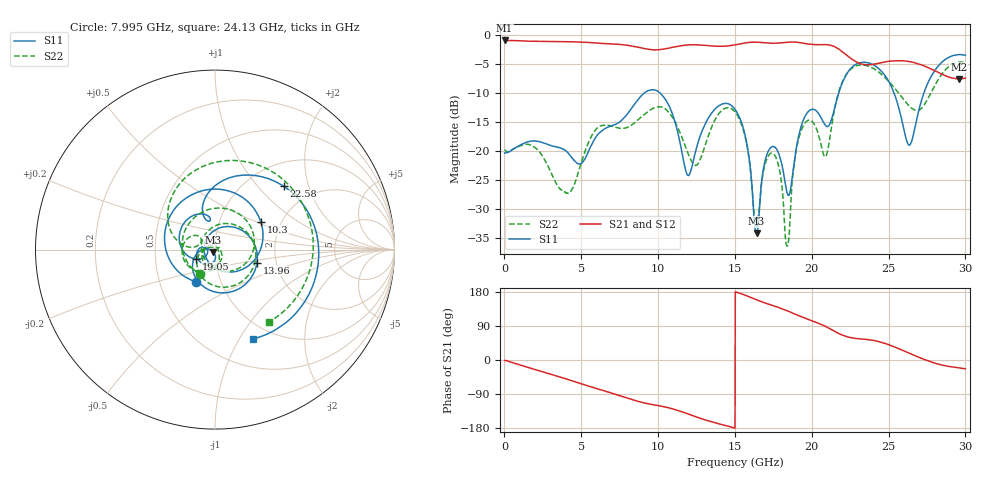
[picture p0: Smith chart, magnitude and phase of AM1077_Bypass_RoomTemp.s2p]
# Hz S DB R 50.0
!freq dBS11 angS11 dBS21 angS21 dBS12 angS12 dBS22 angS22
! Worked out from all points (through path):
!   1601 points, 10 MHz to 30 GHz, reference 50 ohm
!   highest |S21| = -0.94 dB at 10 MHz (marker M1); lowest = -7.6 dB at 29.57 GHz (marker M2)
!   group delay of S21, straight-line fit = 36.5 ps
!   lowest |S11| = -34.3 dB at 16.41 GHz (marker M3), VSWR 1.04, Z = 48.7 - j1.4 ohm
!   |S11| at or under -10 dB: start of sweep to 9.112 GHz; 10.12 GHz to 21.76 GHz (11.64 GHz wide, 73 % of centre); 25.35 GHz to 27.3 GHz (1.946 GHz wide, 7.39 % of centre)
!   |S22| runs from -36.5 to -4.7 dB; largest |S21 - S12| = 0.011
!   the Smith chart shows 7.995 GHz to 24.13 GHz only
!   S11 on the Smith chart (normalised r, x): 7.995 GHz: 0.76, -0.29; 10.3 GHz: 1.58, +0.53; 13.96 GHz: 1.59, -0.24; 19.05 GHz: 0.81, -0.09; 22.58 GHz: 1.44, +1.39; 24.13 GHz: 0.81, -1.14
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1e7  -20.40 -12.1  -0.94 -1.1  -0.91 -0.5  -19.81 -8.3
5.014581e9  -22.17 -167.6  -1.23 -62.9  -1.23 -62.8  -21.92 176.0
7.994838e9  -13.66 -120.2  -1.77 -100.6  -1.79 -100.6  -15.96 -120.6
1.001916e10  -9.79 55.9  -2.55 -120.4  -2.57 -120.3  -12.40 56.9
1.030032e10  -10.51 31.0  -2.46 -122.5  -2.47 -122.5  -12.55 33.8
1.194977e10  -24.27 -173.8  -1.71 -142.4  -1.72 -142.3  -20.49 -103.7
1.395535e10  -12.22 -17.2  -1.95 -168.4  -1.97 -168.3  -13.58 20.9
1.5005e10  -12.85 -97.8  -1.70 -179.8  -1.72 -179.9  -13.27 -75.0
1.641078e10  -34.27 -132.1  -1.24 158.9  -1.26 159.0  -32.99 55.7
1.747918e10  -19.25 -149.6  -1.42 143.4  -1.43 143.4  -20.42 -125.7
1.841636e10  -27.43 179.8  -1.24 129.9  -1.25 129.9  -36.44 48.9
1.905365e10  -18.68 -153.1  -1.25 118.7  -1.26 118.7  -18.97 -97.7
2.000958e10  -12.83 136.2  -1.64 103.4  -1.64 103.5  -14.89 173.7
2.090928e10  -15.68 99.3  -1.66 88.3  -1.67 88.5  -20.97 157.0
2.257748e10  -5.68 42.8  -4.11 58.7  -4.12 58.8  -5.83 75.6
2.413321e10  -5.35 -67.0  -5.00 50.8  -4.99 50.9  -5.97 -52.9
2.501416e10  -8.03 -134.7  -4.54 40.3  -4.54 40.3  -8.01 -130.0
2.634497e10  -19.04 52.1  -4.58 18.0  -4.59 18.1  -12.27 96.9
2.776949e10  -7.16 -131.2  -5.87 -5.2  -5.87 -5.2  -9.94 -84.7
2.874417e10  -4.14 158.5  -7.08 -15.6  -7.09 -15.7  -5.88 -179.1
2.956889e10  -3.39 104.4  -7.58 -20.7  -7.56 -20.6  -4.67 116.6
3e10  -3.48 80.5  -7.46 -23.2  -7.50 -23.2  -4.80 89.6
